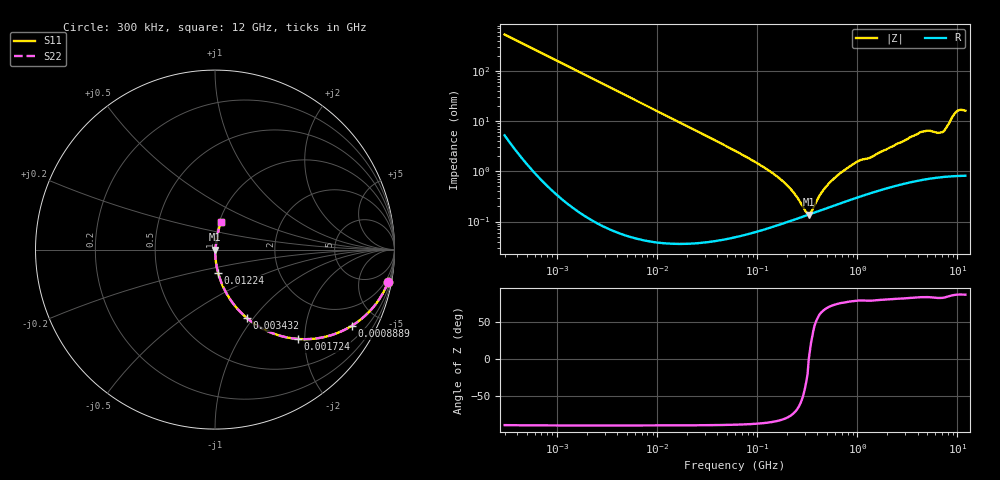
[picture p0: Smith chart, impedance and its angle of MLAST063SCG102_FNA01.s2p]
! MLAST063SCG102_FNA01  S-PARAMETER MODEL  ( General Type )
! Model Generated by TAIYO YUDEN Corporation (http://www.ty-top.com)
! Version 1.0
! TAIYO YUDEN Control No. 160830
! Copyright(c) 2016 TAIYO YUDEN CO.,LTD. All Rights Reserved.
! Product Description (link to TY-COMPAS)
! https://ds.yuden.co.jp/TYCOMPAS/or/detail?pn=MLAST063SCG102JFNA01&u=M
! Products Name : Multilayer Ceramic Capacitors
! Characteristics :
!  Capacitance : 1000 pF , Rated Voltage : 25V , TCC : CG / C0G
!  Case Size : 0.6 x 0.3 / 0.024 x 0.012 [mm/inch] , Thickness : 0.3 / 0.012 [mm/inch]
!  (Conditions: Temperature = 25 degC , DC Bias Current/Voltage = 0A / 0V)
! External Node Assignments :
!  1  o---| |---o  2
! GND o---------o GND
! Frequency Range : 0.3MHz  -  12000MHz  [ 401 STEP ]
# MHz S RI R 50
! Freq[MHz].  S11 Real  S11 Imag  S21 Real  S21 Imag  S12 Real  S12 Imag  S22 Real  S22 Imag
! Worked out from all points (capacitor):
!   401 points, 300 kHz to 12 GHz, reference 50 ohm
!   read as one part in series: C = 1 nF near 316.3 kHz
!   lowest |Z| = 137 mohm at 326.9 MHz (marker M1)
!   series resonance near 327.3 MHz, so ESL is about 240 pH
!   S11 on the Smith chart (normalised r, x): 300 kHz: 1, -11; 888.9 kHz: 1.01, -3.58; 1.724 MHz: 1.00, -1.85; 3.432 MHz: 1.00, -0.93; 12.24 MHz: 1.00, -0.26; 12 GHz: 1.02, +0.32
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0.3  0.964 -0.1814  0.036 0.1814  0.036 0.1814  0.964 -0.1814
0.537322  0.8967 -0.3023  0.1033 0.3023  0.1033 0.3023  0.8967 -0.3023
0.888858  0.7617 -0.4249  0.2383 0.4249  0.2383 0.4249  0.7617 -0.4249
1.723698  0.4603 -0.4976  0.5397 0.4976  0.5397 0.4976  0.4603 -0.4976
1.769972  0.4471 -0.4964  0.5529 0.4964  0.5529 0.4964  0.4471 -0.4964
3.432378  0.1773 -0.3812  0.8227 0.3812  0.8227 0.3812  0.1773 -0.3812
10.44266  0.023 -0.1487  0.977 0.1487  0.977 0.1487  0.023 -0.1487
12.24171  0.0169 -0.1276  0.9831 0.1276  0.9831 0.1276  0.0169 -0.1276
60  0.00114 -0.0256  0.9989 0.0256  0.9989 0.0256  0.00114 -0.0256
173.124  0.000932 -0.00674  0.9991 0.00674  0.9991 0.00674  0.000932 -0.00674
225.6362  0.00107 -0.00386  0.9989 0.00386  0.9989 0.00386  0.00107 -0.00386
301.9711  0.0013 -0.001  0.9987 0.001  0.9987 0.001  0.0013 -0.001
326.9496  0.00137 -9.96e-06  0.9986 9.96e-06  0.9986 9.96e-06  0.00137 -9.96e-06
353.9943  0.00145 0.000849  0.9985 -0.000849  0.9985 -0.000849  0.00145 0.000849
449.3064  0.00173 0.00362  0.9983 -0.00362  0.9983 -0.00362  0.00173 0.00362
651.0506  0.0023 0.00833  0.9977 -0.00833  0.9977 -0.00833  0.0023 0.00833
994.7115  0.00322 0.0152  0.9968 -0.0152  0.9968 -0.0152  0.00322 0.0152
2088.533  0.00555 0.0288  0.9944 -0.0288  0.9944 -0.0288  0.00555 0.0288
4385.161  0.0103 0.0597  0.9897 -0.0597  0.9897 -0.0597  0.0103 0.0597
7064.448  0.0111 0.0587  0.9889 -0.0587  0.9889 -0.0587  0.0111 0.0587
9708.23  0.0301 0.1464  0.9699 -0.1464  0.9699 -0.1464  0.0301 0.1464
12000  0.0327 0.1544  0.9673 -0.1544  0.9673 -0.1544  0.0327 0.1544
